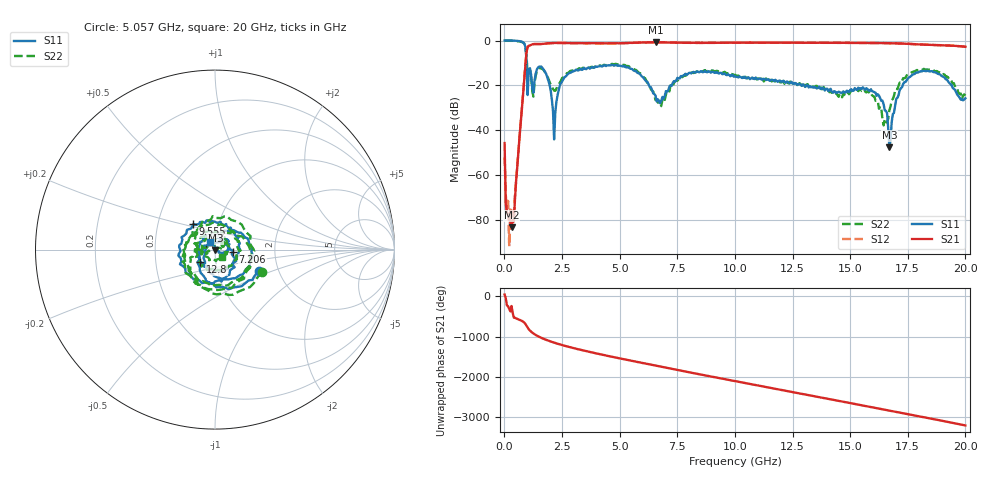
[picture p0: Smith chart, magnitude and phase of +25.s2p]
!Agilent Technologies,E8361C,US49010292,A.09.42.06
!Agilent E8361C: A.09.42.06
!Date: Wednesday, July 09, 2025 01:17:09
!Correction: S11(Full 2 Port(1,2))
!S21(Full 2 Port(1,2))
!S12(Full 2 Port(1,2))
!S22(Full 2 Port(1,2))
!S2P File: Measurements: S11, S21, S12, S22:
# Hz S  dB  R 50
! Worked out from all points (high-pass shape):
!   401 points, 10 MHz to 20 GHz, reference 50 ohm
!   highest |S21| = -0.77 dB at 6.557 GHz (marker M1); lowest = -83.3 dB at 309.9 MHz (marker M2)
!   |S21| within 3 dB of the highest: 988.6 MHz to end of sweep
!   lowest |S11| = -47.6 dB at 16.7 GHz (marker M3), VSWR 1.01, Z = 50.2 - j0.375 ohm
!   |S11| at or under -10 dB: 964.7 MHz to end of sweep
!   |S22| runs from -37.8 to 0.0 dB; largest |S21 - S12| = 0.0085
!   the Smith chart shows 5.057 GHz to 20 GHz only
!   S11 on the Smith chart (normalised r, x): 5.057 GHz: 1.59, -0.40; 7.206 GHz: 1.22, -0.03; 9.555 GHz: 0.76, +0.22; 12.8 GHz: 0.84, -0.12; 20 GHz: 0.94, +0.08
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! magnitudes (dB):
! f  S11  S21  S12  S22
! 10 MHz  0.0  -45.7  -52.1  -0.1
! 159.9 MHz  0.0  -77.5  -71.6  0.0
! 309.9 MHz  0.0  -83.3  -76.1  0.0
! 809.6 MHz  -0.8  -24.1  -24.1  -0.9
! 1.059 GHz  -12.7  -2.4  -2.4  -13.0
! 1.709 GHz  -13.1  -1.4  -1.5  -13.2
! 2.159 GHz  -44.1  -1.1  -1.1  -22.3
! 2.509 GHz  -18.2  -1.1  -1.1  -16.6
! 3.358 GHz  -13.1  -1.2  -1.1  -12.5
! 5.057 GHz  -11.3  -1.2  -1.2  -10.8
! 6.557 GHz  -24.6  -0.8  -0.8  -26.6
! 6.707 GHz  -26.8  -0.8  -0.8  -28.0
! 7.206 GHz  -20.0  -0.9  -0.9  -20.2
! 9.555 GHz  -14.6  -1.0  -1.0  -14.0
! 10.01 GHz  -16.0  -1.0  -1.0  -15.3
! 12.8 GHz  -19.4  -1.0  -1.0  -19.0
! 13.35 GHz  -20.7  -1.0  -1.0  -20.4
! 16 GHz  -22.8  -1.1  -1.1  -24.8
! 16.7 GHz  -47.6  -1.2  -1.2  -31.2
! 17.25 GHz  -20.8  -1.4  -1.3  -18.1
! 17.95 GHz  -14.2  -1.7  -1.7  -13.4
! 20 GHz  -25.8  -2.8  -2.8  -24.6
